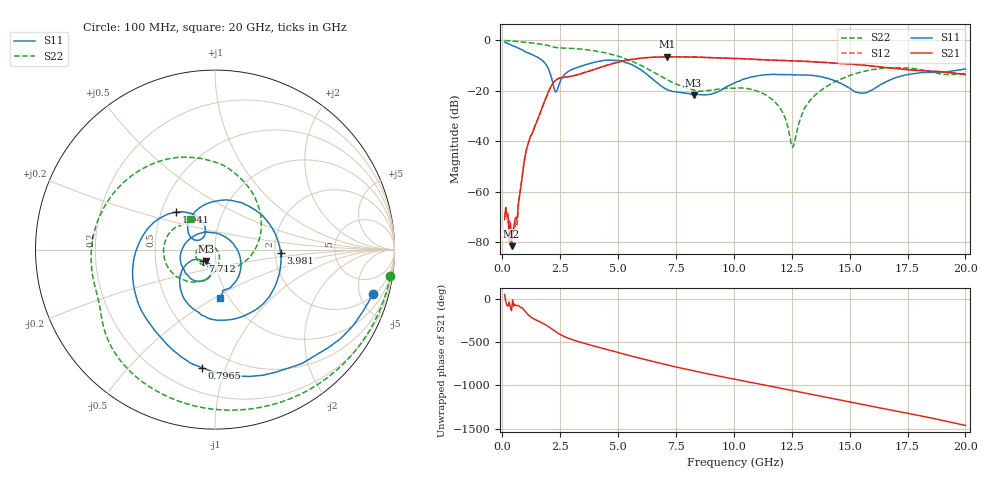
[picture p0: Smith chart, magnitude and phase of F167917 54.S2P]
!  2-Port S-parameters saved by WinCal
! VAR MeasName=S-Parameters (CALIBRATED_DATA) read from VNA (N5242A)
! VAR MeasDate=2016-11-22 9:02:36
! VAR NAME=F167917 54
! VAR FILENAME=F167917 54.S2P
! VAR DATE=2016-11-22 9:02:36
! VAR PHYS_PORTS=1,2
# Hz S DB R 50
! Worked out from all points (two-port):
!   401 points, 100 MHz to 20 GHz, reference 50 ohm
!   highest |S21| = -6.56 dB at 7.115 GHz (marker M1); lowest = -81.5 dB at 398.5 MHz (marker M2)
!   |S21| within 3 dB of the highest: 4.641 GHz to 15.24 GHz (10.6 GHz wide, 107 % of centre)
!   lowest |S11| = -21.7 dB at 8.259 GHz (marker M3), VSWR 1.18, Z = 44.9 - j5.94 ohm
!   |S11| at or under -10 dB: 1.913 GHz to 3.5 GHz (1.588 GHz wide, 58.7 % of centre); 5.668 GHz to end of sweep
!   |S22| runs from -42.4 to -0.1 dB; largest |S21 - S12| = 0.0048
!   S11 on the Smith chart (normalised r, x): 100 MHz: 2.18, -6.62; 796.5 MHz: 0.36, -0.83; 1.941 GHz: 0.60, +0.27; 3.981 GHz: 2.15, -0.10; 7.712 GHz: 0.87, -0.11; 20 GHz: 0.91, -0.53
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1e8  -0.77 -15.5  -70.99 45.8  -70.17 56.6  -0.10 -8.7
3.985e8  -1.95 -52.6  -81.53 -140.4  -79.42 -117.5  -0.29 -32.9
5.4775e8  -2.51 -69.2  -71.05 -66.4  -74.85 -57.8  -0.40 -44.6
7.965e8  -3.58 -96.2  -58.31 -107.0  -58.62 -102.3  -0.63 -63.3
1.095e9  -4.99 -126.2  -41.65 178.6  -41.59 179.2  -0.92 -84.1
1.94075e9  -10.41 136.0  -21.57 45.2  -21.54 45.3  -2.00 -136.1
2.33875e9  -20.33 143.5  -15.63 -28.4  -15.60 -28.3  -2.92 -154.2
3.43325e9  -10.22 49.9  -13.18 -148.9  -13.16 -148.9  -3.56 160.3
3.9805e9  -8.72 -3.1  -11.55 170.1  -11.53 170.3  -4.21 136.2
5.3735e9  -8.95 -107.3  -7.90 70.3  -7.83 70.2  -7.53 69.8
6.7665e9  -17.43 -154.9  -6.62 -24.0  -6.62 -24.1  -13.82 -9.1
7.11475e9  -19.54 -148.4  -6.56 -46.0  -6.57 -46.1  -15.59 -30.1
7.71175e9  -20.71 -136.5  -6.61 -82.2  -6.62 -82.1  -18.03 -64.9
8.259e9  -21.66 -127.3  -6.63 -114.0  -6.62 -113.9  -19.73 -92.9
1.005e10  -16.87 -100.1  -7.23 147.2  -7.22 147.3  -19.01 -146.2
1.17415e10  -13.51 -131.5  -7.94 58.6  -7.89 58.5  -24.07 153.8
1.25375e10  -13.71 -145.3  -8.18 17.6  -8.16 17.2  -42.43 47.3
1.338325e10  -13.95 -164.1  -8.52 -27.5  -8.50 -27.6  -22.89 -71.3
1.55225e10  -20.97 69.0  -9.83 -140.6  -9.88 -140.7  -12.55 -131.8
1.67165e10  -15.84 -26.7  -10.92 156.3  -10.94 156.9  -10.89 -167.2
1.8209e10  -12.77 -71.0  -12.11 78.5  -12.00 78.7  -11.89 151.6
2e10  -11.37 -83.8  -13.64 -24.8  -13.53 -24.9  -13.22 128.8
